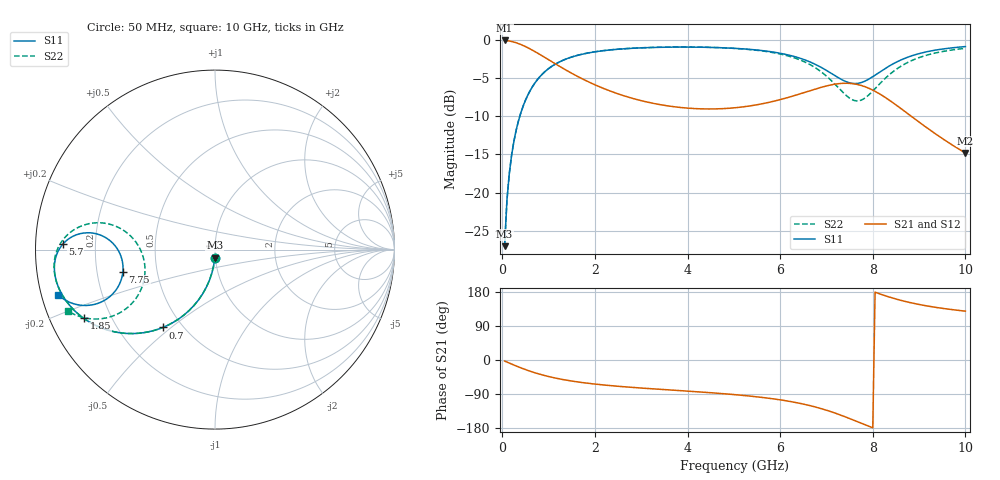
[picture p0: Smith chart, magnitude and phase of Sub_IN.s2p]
! Created Wed Jul 11 12:19:22 2018
# ghz S ma R 50
! 2 Port Network Data from SP1.SP block
! freq  magS11  angS11  magS21  angS21  magS12  angS12  magS22  angS22
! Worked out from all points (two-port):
!   200 points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, 50 MHz to 10 GHz, reference 50 ohm
!   highest |S21| = -0.02 dB at 50 MHz (marker M1); lowest = -14.8 dB at 10 GHz (marker M2)
!   |S21| within 3 dB of the highest: start of sweep to 1.126 GHz
!   lowest |S11| = -27.0 dB at 50 MHz (marker M3), VSWR 1.09, Z = 49.7 - j4.43 ohm
!   |S11| at or under -10 dB: start of sweep to 377.5 MHz
!   |S22| runs from -27.0 to -0.9 dB; largest |S21 - S12| = 0
!   S11 on the Smith chart (normalised r, x): 50 MHz: 0.99, -0.09; 700 MHz: 0.39, -0.47; 1.85 GHz: 0.10, -0.24; 5.7 GHz: 0.08, +0.02; 7.75 GHz: 0.31, -0.11; 10 GHz: 0.05, -0.14
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0.05  0.04445 -91.1  0.9977 -2.7  0.9977 -2.7  0.04444 -91.1
0.1  0.08859 -94.6  0.9946 -5.4  0.9946 -5.4  0.08858 -94.6
0.15  0.1322 -97.6  0.9896 -8.0  0.9896 -8.0  0.1321 -97.6
0.25  0.2166 -103.1  0.9739 -13.2  0.9739 -13.2  0.2166 -103.0
0.45  0.3694 -113.1  0.9248 -23.0  0.9248 -23.0  0.3695 -113.1
0.7  0.5223 -123.8  0.8447 -33.5  0.8447 -33.5  0.5223 -123.8
1.2  0.7125 -139.7  0.6848 -49.0  0.6848 -49.0  0.7128 -139.7
1.75  0.8137 -150.8  0.554 -59.9  0.554 -59.9  0.8143 -150.9
1.85  0.8253 -152.4  0.5355 -61.4  0.5355 -61.4  0.8261 -152.4
2.5  0.8739 -160.3  0.4449 -69.3  0.4449 -69.3  0.8749 -160.5
3.4  0.8997 -167.8  0.3783 -77.3  0.3783 -77.3  0.9007 -168.1
5.05  0.8845 -177.9  0.3611 -91.7  0.3611 -91.7  0.8835 -179.2
5.7  0.8495 178.0  0.3877 -100.1  0.3877 -100.1  0.8445 175.9
6.25  0.7909 174.5  0.4283 -110.2  0.4283 -110.2  0.7769 171.0
6.7  0.7087 172.4  0.4724 -122.1  0.4724 -122.1  0.6777 167.3
7.2  0.5819 175.5  0.516 -140.7  0.516 -140.7  0.5087 168.7
7.55  0.5218 -174.2  0.5198 -157.0  0.5198 -157.0  0.4081 -177.4
7.75  0.5277 -166.5  0.5051 -166.8  0.5051 -166.8  0.4047 -164.5
8  0.577 -159.1  0.4708 -178.8  0.4708 -178.8  0.4644 -152.0
8.35  0.6762 -155.3  0.4057 166.4  0.4057 166.4  0.5918 -146.4
8.95  0.8097 -157.5  0.2979 147.7  0.2979 147.7  0.7599 -149.4
10  0.9095 -163.9  0.1819 128.9  0.1819 128.9  0.886 -157.2
